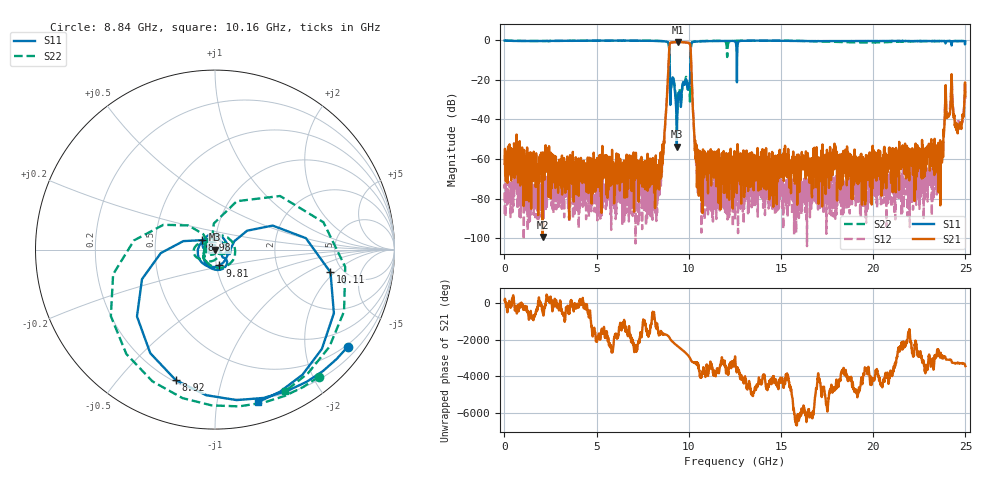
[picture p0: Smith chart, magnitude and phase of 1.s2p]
! 2/28/2023 11:29:43 AM
! D:\_XLC\ZBF16-C9.5-1G-340\1.S2P
! CHANNEL.1
! TR.MEASUREMENT
! CORRECTED.DATA
! RF.CORRECTION: FULL.TWO.PORT.CAL.PORT.1.2
! AVERAGING.OFF
! IF.BANDWIDTH: 100KHZ
! SWEEPTYPE:  FREQ.SWEEP(Linear)
! Reference Plane Port Info
! PORT:  PORT1  PORT2
! DISTANCE:  0  m  0  m
! TIME:  0  s  0  s
! PHASE.OFFSET:  0 °  0 °
! LOSS:  0  dB  0  dB
! REF.LOSS:  0  dB  0  dB
! REF.FREQ:  0  Hz  0  Hz
! Power Info
! POWER:  0  dBm  0  dBm
! EFF.POWER:  -10  dBm  0  dBm
! SOURCE.ATTEN:  10  dB  0  dB
! TEST.ATTEN:  0  dB  0  dB
# GHZ S RI R 50.0
! FREQ.GHZ  S11RE  S11IM  S21RE  S21IM  S12RE  S12IM  S22RE  S22IM
!; PortSelection: Port_12
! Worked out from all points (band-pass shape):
!   2500 points, 10 MHz to 25 GHz, reference 50 ohm
!   highest |S21| = -0.80 dB at 9.41 GHz (marker M1); lowest = -99.5 dB at 2.07 GHz (marker M2)
!   |S21| within 3 dB of the highest: 8.943 GHz to 10.09 GHz (1.152 GHz wide, 12.1 % of centre)
!   lowest |S11| = -53.7 dB at 9.35 GHz (marker M3), VSWR 1.00, Z = 50.2 + j0.0104 ohm
!   |S11| at or under -10 dB: 8.959 GHz to 10.09 GHz (1.129 GHz wide, 11.9 % of centre); 12.5964 GHz to 12.61887 GHz (22.47 MHz wide, 0.178 % of centre)
!   |S22| runs from -40.5 to 0.0 dB; largest |S21 - S12| = 0.041
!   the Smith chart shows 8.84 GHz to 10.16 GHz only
!   S11 on the Smith chart (normalised r, x): 8.84 GHz: 0.44, -3.00; 8.92 GHz: 0.21, -0.72; 8.98 GHz: 0.86, +0.09; 9.81 GHz: 1.03, -0.18; 10.11 GHz: 3.98, -1.77; 10.16 GHz: 0.17, -1.31
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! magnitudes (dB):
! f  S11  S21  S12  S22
! 10 MHz  0.0  -62.4  -87.9  0.0
! 2.07 GHz  -0.3  -99.5  -77.7  -0.3
! 4.18 GHz  -0.1  -68.3  -77.2  -0.2
! 8.34 GHz  -0.2  -72.1  -75.8  -0.2
! 8.84 GHz  -0.8  -23.4  -24.4  -0.8
! 8.92 GHz  -2.4  -8.1  -7.8  -2.4
! 8.98 GHz  -20.9  -1.4  -1.4  -19.3
! 9.35 GHz  -53.7  -0.8  -0.8  -40.5
! 9.41 GHz  -29.9  -0.8  -0.8  -29.0
! 9.81 GHz  -20.7  -1.0  -1.0  -20.2
! 10.11 GHz  -3.7  -6.6  -6.3  -4.1
! 10.16 GHz  -1.1  -19.8  -20.1  -1.1
! 10.37 GHz  -0.6  -60.0  -59.7  -0.5
! 10.6 GHz  -0.5  -62.7  -77.1  -0.3
! 12.51 GHz  -0.5  -62.0  -90.6  -0.1
! 16.67 GHz  -0.3  -77.3  -82.4  -0.4
! 20.84 GHz  -0.3  -58.9  -67.4  -0.8
! 23.33 GHz  -0.3  -49.8  -70.4  -0.3
! 23.66 GHz  -0.3  -57.5  -60.6  -0.3
! 23.97 GHz  -0.4  -35.6  -34.7  -0.3
! 24.67 GHz  -0.3  -43.1  -43.2  -0.4
! 25 GHz  -0.5  -28.1  -29.5  -0.4
